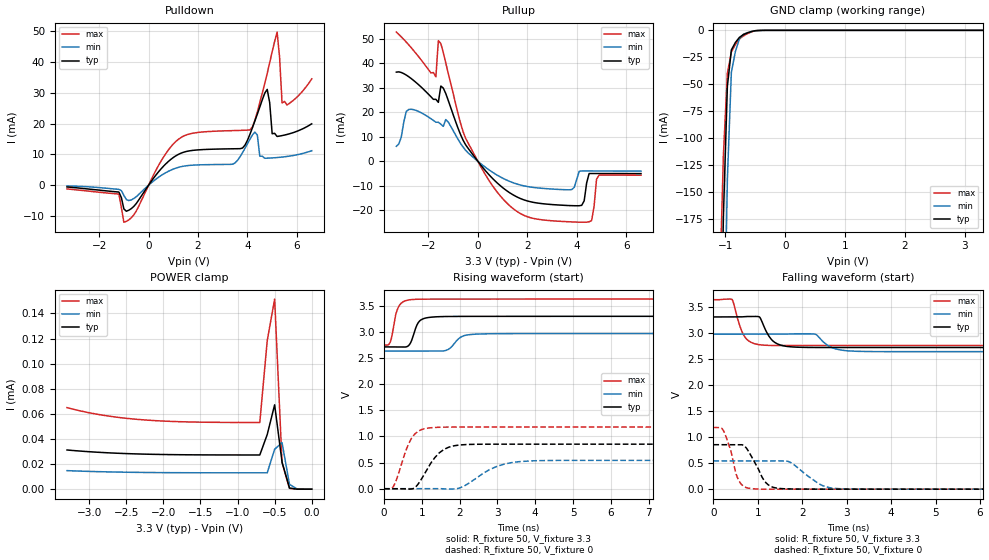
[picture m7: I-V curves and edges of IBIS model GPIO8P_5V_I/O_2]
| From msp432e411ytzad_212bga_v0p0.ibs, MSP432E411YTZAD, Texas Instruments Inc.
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|   Model Cell GPIO8P_5V_I/O_2
[Model]   GPIO8P_5V_I/O_2
Model_type   I/O
Polarity   Non-Inverting
Enable   Active-Low
Vinl =  0.8
Vinh =  2
Cref =  15.0000pF
Rref =  100.0000M
Vref =  0V
Vmeas =  1.65
C_comp   7.738177p   6.063161p   9.392973p
[Model Spec]
Vinl   0.8   0.8   0.8
Vinh   2   2   2
[Temperature Range]   25   125   -40
[Voltage Range]   3.3   2.97   3.63
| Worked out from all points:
|   slope of the pulldown table from 0 to 0.495 V, typ, clamps not added: 95.1 ohm
|   slope of the pullup table from 0 to 0.495 V, typ, clamps not added: 83.2 ohm
|   GND clamp passes 1 mA (typ) near -0.55 V on its own axis
|   rising waveform, R_fixture 50, V_fixture 3.3: 20-80 % time 183ps typ, 267ps min, 156ps max; typ from 2.71 V to 3.3 V
|   rising waveform, R_fixture 50, V_fixture 0: 20-80 % time 477ps typ, 760ps min, 352ps max; typ from 0 V to 0.852 V
|   falling waveform, R_fixture 50, V_fixture 3.3: 20-80 % time 246ps typ, 318ps min, 212ps max; typ from 3.3 V to 2.71 V
|   falling waveform, R_fixture 50, V_fixture 0: 20-80 % time 318ps typ, 502ps min, 225ps max; typ from 0.852 V to 0 V
| Nom Voltages:
|   VDDC=1.2, VDD=3.3, GND=0
| Min Voltages:
|   VDDC=1.08, VDD=2.97, GND=0
| Max Voltages:
|   VDDC=1.32, VDD=3.63, GND=0
[POWER_clamp]
|   voltage   I(typ)   I(min)   I(max)
-3.3V     31.22uA    14.77uA    64.95uA
-2.8V     29.13uA    13.84uA    58.77uA
-2.3V     27.98uA    13.34uA    55.36uA
-1.7V     27.4uA     13.1uA     53.62uA
-700mV    27.24uA    13.03uA    53.12uA
-600mV    43.52uA    13.03uA    118.2uA
-500mV    67.2uA     31.8uA     151.5uA
-400mV    21.58uA    37.04uA    21.1uA
-300mV    927.4nA    3.873uA    611.4nA
-200mV    28.93nA    266.5nA    11.51nA
0V        696.9pA    10.99nA    568.3pA
[Pulldown]
|   voltage   I(typ)   I(min)   I(max)
-3.3V     -580.7uA   -252.6uA   -1.206mA
-1.2V     -2.224mA   -1.36mA    -2.903mA
-1V       -7.701mA   -3.323mA   -12.01mA
1.2V      9.981mA    5.78mA     14.86mA
3.4V      11.82mA    6.814mA    17.72mA
4.1V      16.51mA    14.91mA    17.95mA
4.3V      20.83mA    17.22mA    21.06mA
4.8V      31.11mA    8.778mA    36.31mA
5V        16.71mA    8.862mA    43.35mA
5.2V      15.82mA    8.977mA    49.72mA
5.4V      16.11mA    9.128mA    26.68mA
6.6V      19.93mA    11.19mA    34.53mA
[Pullup]
|   voltage   I(typ)   I(min)   I(max)
-3.3V     36.34mA    6.118mA    52.65mA
-2.8V     34.47mA    21.12mA    47.47mA
-1.7V     25.26mA    15.93mA    34.41mA
-1.6V     24.03mA    15.9mA     49.16mA
-1.5V     30.66mA    15.13mA    48.01mA
-500mV    6.804mA    4.54mA     9.445mA
1.7V      -15.06mA   -9.595mA   -21.16mA
3.8V      -18.05mA   -11.48mA   -24.67mA
4.2V      -17.92mA   -3.913mA   -24.78mA
4.5V      -4.967mA   -3.92mA    -24.61mA
4.9V      -4.967mA   -3.932mA   -5.627mA
6.6V      -5.001mA   -3.99mA    -5.632mA
[GND_clamp]
|   voltage   I(typ)   I(min)   I(max)
-3.3V     -16.36A    -15.34A    -17.18A
-1.1V     -382.1mA   -633.4mA   -250.1mA
-1.033V   -173.3mA   -336.5mA   -116.4mA
-966.7mV  -52.02mA   -138.4mA   -39.81mA
-900mV    -18.21mA   -38.98mA   -20.34mA
-833.3mV  -11.36mA   -19.82mA   -13.17mA
-766.7mV  -6.618mA   -8.051mA   -8.134mA
-700mV    -3.983mA   -3.675mA   -5.247mA
-500mV    -328.3uA   -388.2uA   -374.5uA
-366.7mV  -15.94uA   -32.84uA   -14.83uA
3.3V      697pA      8.348uA    426.1pA
[Ramp]
| variable   typ   min   max
dV/dt_f 0.35736481/0.24671888n 0.20491811/0.31942174n 0.53454654/0.21282663n
dV/dt_r 0.51638227/0.48110981n 0.32917821/0.76593586n 0.71404066/0.35410299n
R_load = 50
[Rising Waveform]
R_fixture = 50
V_fixture = 3.3
V_fixture_min = 2.97
V_fixture_max = 3.63
|   time   V(typ)   V(min)   V(max)
0s        2.714V     2.635V     2.751V
173.5ps   2.714V     2.635V     2.827V
391.7ps   2.715V     2.635V     3.494V
647.3ps   2.739V     2.635V     3.612V
779.1ps   2.946V     2.635V     3.624V
975.6ps   3.232V     2.635V     3.628V
1.544ns   3.295V     2.635V     3.629V
2.099ns   3.299V     2.925V     3.63V
2.578ns   3.299V     2.963V     3.63V
20.01ns   3.3V       2.97V      3.63V
[Rising Waveform]
R_fixture = 50
V_fixture = 0
V_fixture_min = 0
V_fixture_max = 0
|   time   V(typ)   V(min)   V(max)
0s        0V         0V         0V
268.7ps   0V         0V         70.61mV
633.8ps   -7.379mV   0V         836.1mV
806.6ps   17.89mV    0V         1.043V
1.302ns   556.6mV    0V         1.171V
1.588ns   753.6mV    -3.772mV   1.178V
1.844ns   820.9mV    -5.398mV   1.18V
2.991ns   852.2mV    429.1mV    1.181V
3.843ns   852.1mV    531.2mV    1.181V
20.02ns   852.2mV    541.8mV    1.181V
[Falling Waveform]
R_fixture = 50
V_fixture = 3.3
V_fixture_min = 2.97
V_fixture_max = 3.63
|   time   V(typ)   V(min)   V(max)
0s        3.3V       2.97V      3.63V
419.1ps   3.3V       2.97V      3.635V
714.6ps   3.307V     2.97V      2.907V
1.036ns   3.299V     2.97V      2.768V
1.18ns    3.039V     2.97V      2.757V
1.436ns   2.785V     2.97V      2.752V
1.986ns   2.717V     2.976V     2.752V
2.733ns   2.715V     2.692V     2.752V
3.263ns   2.714V     2.641V     2.752V
20.01ns   2.714V     2.635V     2.752V
[Falling Waveform]
R_fixture = 50
V_fixture = 0
V_fixture_min = 0
V_fixture_max = 0
|   time   V(typ)   V(min)   V(max)
0s        852.2mV    541.8mV    1.181V
237.5ps   852.2mV    541.8mV    1.101V
591ps     853.4mV    541.8mV    135.9mV
720.8ps   808.6mV    541.8mV    36.25mV
899.5ps   559mV      541.8mV    6.651mV
1.225ns   89.02mV    541.8mV    0V
1.68ns    4.723mV    531.8mV    0V
2.39ns    0V         96.08mV    0V
2.871ns   0V         7.909mV    0V
20.02ns   0V         0V         0V
